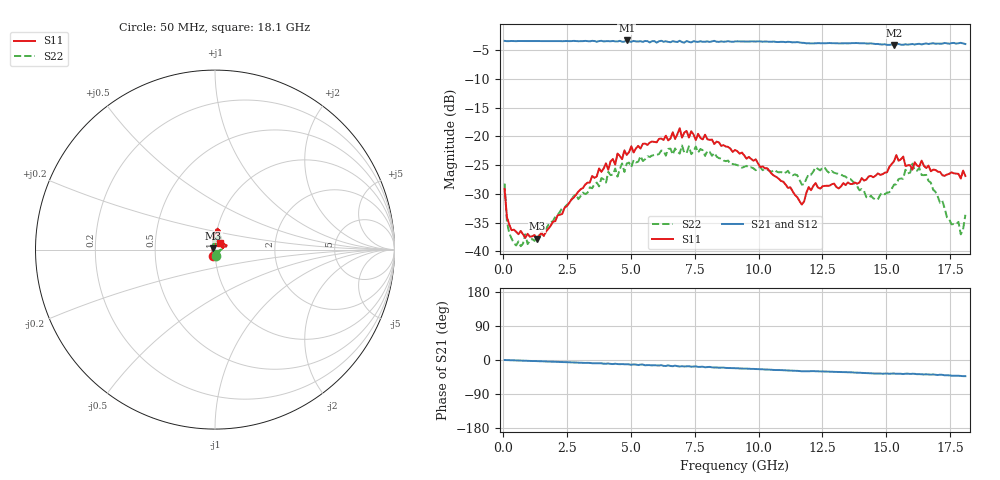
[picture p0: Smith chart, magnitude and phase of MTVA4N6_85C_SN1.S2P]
! Network Analyzer HP8720D.06.14 Serial No. US36140669
! 28 Jun 2005  13:56:45
! Frequency  S11  S21  S12  S22
# HZ  S  DB R 50
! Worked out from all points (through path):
!   201 points, 50 MHz to 18.1 GHz, reference 50 ohm
!   highest |S21| = -3.32 dB at 4.833 GHz (marker M1); lowest = -4.1 dB at 15.3 GHz (marker M2)
!   group delay of S21, straight-line fit = 6.57 ps
!   lowest |S11| = -37.8 dB at 1.313 GHz (marker M3), VSWR 1.03, Z = 49 + j0.785 ohm
!   |S11| at or under -10 dB: start of sweep to end of sweep
!   |S22| runs from -39.1 to -21.6 dB; largest |S21 - S12| = 0.021
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5e7  -29.12 -107.3  -3.39 -0.1  -3.43 0.2  -28.20 -81.0
1.4025e8  -34.05 -131.9  -3.44 -0.2  -3.44 -0.2  -34.84 -119.7
4.11e8  -36.23 -168.1  -3.43 -1.0  -3.43 -1.0  -38.54 -157.0
1.3135e9  -37.78 141.7  -3.43 -3.0  -3.43 -2.9  -37.49 142.9
3.1185e9  -28.99 82.4  -3.44 -7.1  -3.45 -7.4  -29.77 106.6
4.83325e9  -23.23 80.2  -3.32 -11.2  -3.42 -11.8  -24.72 83.1
6.09675e9  -20.45 76.9  -3.46 -14.5  -3.41 -14.5  -23.08 77.9
6.909e9  -18.58 83.0  -3.37 -17.2  -3.46 -16.4  -23.00 69.1
7.54075e9  -20.64 79.8  -3.52 -16.8  -3.41 -18.4  -21.76 74.3
9.075e9  -22.38 95.7  -3.49 -21.6  -3.48 -21.7  -24.89 54.2
1.115075e10  -28.97 95.6  -3.55 -27.6  -3.58 -27.9  -25.99 38.7
1.169225e10  -31.86 99.7  -3.72 -29.7  -3.72 -29.7  -28.39 46.9
1.21435e10  -28.61 87.7  -3.83 -29.3  -3.80 -29.6  -26.09 57.9
1.3407e10  -28.48 50.6  -3.82 -32.1  -3.79 -32.3  -27.00 52.5
1.43095e10  -26.98 14.2  -3.86 -34.8  -3.82 -35.1  -30.74 59.5
1.512175e10  -25.30 24.1  -4.09 -36.2  -4.02 -36.0  -29.72 73.1
1.530225e10  -24.34 19.4  -4.10 -35.6  -4.01 -36.7  -28.40 73.7
1.566325e10  -23.51 17.6  -4.06 -37.1  -4.00 -36.2  -27.37 54.9
1.602425e10  -25.80 25.9  -3.94 -36.4  -4.06 -37.7  -24.75 39.8
1.638525e10  -24.22 32.1  -4.02 -37.6  -3.85 -37.5  -26.73 23.9
1.79195e10  -27.34 56.8  -3.73 -42.2  -3.65 -41.6  -37.04 -56.3
1.81e10  -26.89 52.0  -3.94 -42.7  -3.93 -43.4  -33.64 -71.3
